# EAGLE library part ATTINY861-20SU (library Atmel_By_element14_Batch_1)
8-bit Microcontroller with In-System Programmable Flash
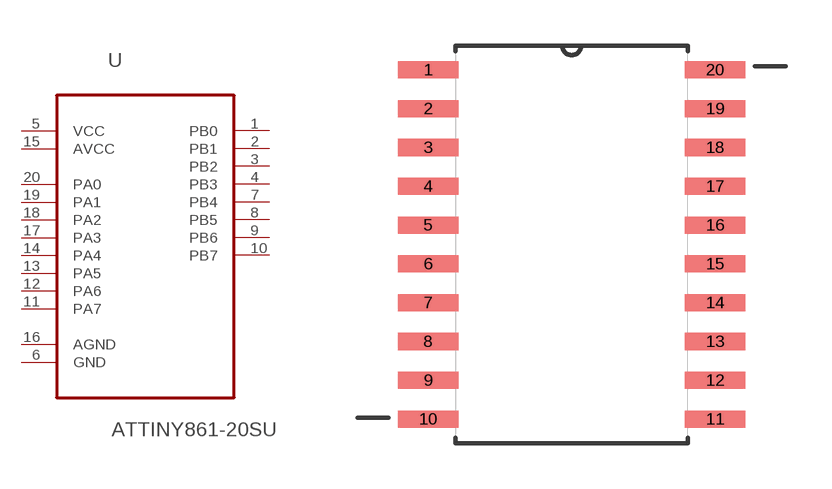
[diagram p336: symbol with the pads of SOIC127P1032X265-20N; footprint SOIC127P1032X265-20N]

Designator prefix U

## ATTINY861-20SU (MPN: ATTINY861-20SU; OC_FARNELL: 1455168; OC_NEWARK: 58M3801; PACKAGE: SOIC-20; SUPPLIER: Atmel)  [SOIC127P1032X265-20N]
1  PB0
2  PB1
3  PB2
4  PB3
5  VCC  pwr
6  GND  pas
7  PB4
8  PB5
9  PB6
10  PB7
11  PA7
12  PA6
13  PA5
14  PA4
15  AVCC  pwr
16  AGND  pas
17  PA3
18  PA2
19  PA1
20  PA0

## Footprint SOIC127P1032X265-20N (pad centres in mm)
smd 1.981 x 0.559: 1 -4.699,5.715; 2 -4.699,4.445; 3 -4.699,3.175; 4 -4.699,1.905; 5 -4.699,0.635; 6 -4.699,-0.635; 7 -4.699,-1.905; 8 -4.699,-3.175; 9 -4.699,-4.445; 10 -4.699,-5.715; 11 4.699,-5.715; 12 4.699,-4.445; 13 4.699,-3.175; 14 4.699,-1.905; 15 4.699,-0.635; 16 4.699,0.635; 17 4.699,1.905; 18 4.699,3.175; 19 4.699,4.445; 20 4.699,5.715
